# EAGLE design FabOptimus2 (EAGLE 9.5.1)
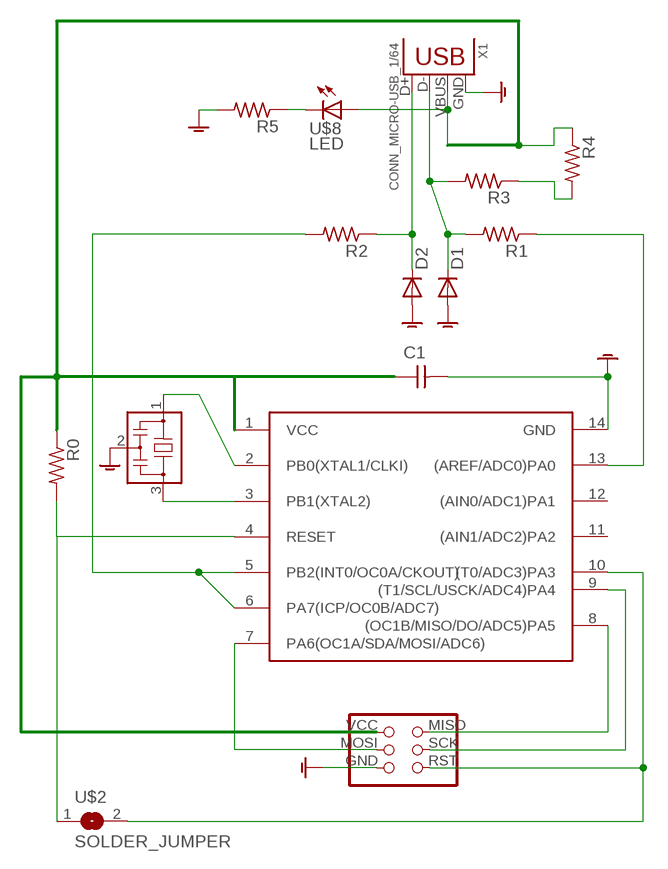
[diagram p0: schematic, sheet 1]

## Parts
C1  CAP-UNPOLARIZEDFAB  [C1206FAB]
D1  DIODESOD123  [SOD123]
D2  DIODESOD123  [SOD123]
IC1  ATTINY44-SSU  [SOIC14_ATTTINY44]
JP1  2X3PINHEADER  [2X3PINHEADER]
R0  RES-US1206FAB  [R1206FAB]
R1  RES-US1206FAB  [R1206FAB]
R2  RES-US1206FAB  [R1206FAB]
R3  RES-US1206FAB  [R1206FAB]
R4  RES-US1206FAB  [R1206FAB]
R5  RES-US1206  [R1206]
U$1  RESONATOR  [EFOBM]
U$2  SOLDER_JUMPER  [SOLDERJUMPER]
U$8  LED  [LED1206]
X1  CONN_MICRO-USB_1/64  [DX4R005HJ5_64]

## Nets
GND: C1.2 D1.ANODE(A) D2.ANODE(A) IC1.14(GND) JP1.GND R5.2 U$1.2 X1.GND
N$1: IC1.2(PB0(XTAL1/CLKI)) U$1.1
N$2: D2.CATHODE(C) R2.1 X1.D+
N$3: IC1.9((T1/SCL/USCK/ADC4)PA4) JP1.SCK
N$4: D1.CATHODE(C) R1.2 R3.2 X1.D-
N$5: IC1.7(PA6(OC1A/SDA/MOSI/ADC6)) JP1.MOSI
N$6: IC1.5(PB2(INT0/OC0A/CKOUT)) IC1.6(PA7(ICP/OC0B/ADC7)) R2.2
N$7: IC1.3(PB1(XTAL2)) U$1.3
N$8: IC1.13((AREF/ADC0)PA0) R1.1
N$9: IC1.8((OC1B/MISO/DO/ADC5)PA5) JP1.MISO
N$10: IC1.10((T0/ADC3)PA3) JP1.RST U$2.2
N$11: IC1.4(RESET) R0.2 U$2.1
N$12: R3.1 R4.2
N$14: R5.1 U$8.2(C)
R4: C1.1 IC1.1(VCC) JP1.VCC R0.1 R4.1 U$8.1(A) X1.VBUS
Unconnected: IC1.11((AIN1/ADC2)PA2) IC1.12((AIN0/ADC1)PA1)

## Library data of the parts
C1 = fab:CAP-UNPOLARIZED
D1 D2 = fab:DIODE: DIODE
IC1 = myFab:ATTINY44
JP1 = myFab:2X3PINHEADER: PIN HEADER
R0 R1-R5 = fab:RES-US: Resistor (US Symbol)
U$1 = fab:RESONATOR
U$2 = myFab:SOLDER_JUMPER
U$8 = fab:LED: LED
X1 = fab:CONN_MICRO-USB: SMD micro USB connector as found in the fablab inventory. Three footprint variants included: original, as described by manufacturer's datasheet for milling with the 1/100" bit for milling with the 1/64" bit Made by Zaerc.

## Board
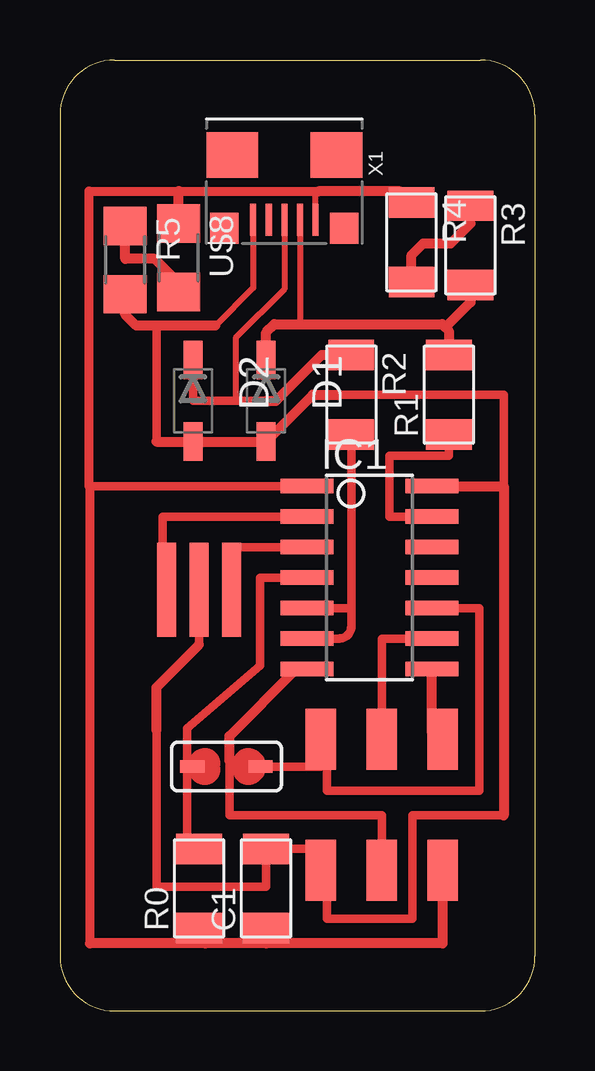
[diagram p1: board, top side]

Size 19.81 x 39.62 mm. Coordinates in mm from the lower left corner, seen from the top.
Outline: 2.29,39.62 17.53,39.62 arc-90 19.81,37.34 19.81,2.29 arc-90 17.53,0 2.29,0 arc-90 0,2.29 0,37.34 arc-90 2.29,39.62
Copper layers (1*16): Top 0.035mm / dielectric 1.5mm / Bottom 0.035mm
Design rules "default *": minimum track width 10mil, minimum drill 24mil, track to track 16mil, track to pad 16mil, pad to pad 16mil, via to via 16mil, smd to smd 16mil, copper to edge 40mil, drill to drill 8mil, minimum pad ring 10mil, minimum via ring 8mil, stop-mask expansion 4mil, vias tented up to drill 0mil, thermal gap 10mil

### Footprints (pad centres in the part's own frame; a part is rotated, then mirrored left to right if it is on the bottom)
C1206FAB = smd 1.27 x 1.905: 1 -1.651,0; 2 1.651,0
SOD123 = smd 1.6 x 0.8: ANODE 1.7,0; CATHODE -1.7,0
SOIC14_ATTTINY44 = smd 2.21 x 0.61: 1 -3.873,3.81; 2 -3.873,2.54; 3 -3.873,1.27; 4 -3.873,0; 5 -3.873,-1.27; 6 -3.873,-2.54; 7 -3.873,-3.81; 8 1.333,-3.81; 9 1.333,-2.54; 10 1.333,-1.27; 11 1.333,0; 12 1.333,1.27; 13 1.333,2.54; 14 1.333,3.81
2X3PINHEADER = smd 2.54 x 1.27: GND -2.54,2.54; MISO 2.92,-2.54; MOSI -2.54,0; RST 2.92,2.54; SCK 2.92,0; VCC -2.54,-2.54
R1206FAB = smd 1.27 x 1.905: 1 -1.651,0; 2 1.651,0
R1206 = smd 1.6 x 1.803: 1 -1.422,0; 2 1.422,0
EFOBM = smd 0.8 x 3.9: 1 -1.35,0; 2 0,0; 3 1.35,0
SOLDERJUMPER = smd 1.016 x 0.508: 1 -2.057,0; 2 0.787,0
LED1206 = smd 1.6 x 1.803: 1 -1.422,0; 2 1.422,0
DX4R005HJ5_64 = smd 0.254 x 1.35: D+ 0,1.6; D- -0.65,1.6; GND 1.3,1.6; ID 0.65,1.6; VBUS -1.3,1.6 | smd 1.2 x 1.3: GND@1 -2.5,1.95; GND@2 2.5,1.95 | smd 2.15 x 1.9: GND@3 -2.175,-1.1; GND@4 2.175,-1.1

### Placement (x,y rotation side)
C1  8.6,5.11 90 top
D1  8.6,25.43 270 top
D2  5.55,25.43 270 top
IC1  14.18,18.06 0 top
JP1  13.42,8.41 90 top
R0  5.8,5.11 90 top
R1  16.22,25.68 90 top
R2  12.15,25.68 270 top
R3  17.12,31.9 270 top
R4  14.66,32.03 270 top
R5  2.72,31.29 270 top
U$1  5.8,17.55 0 top
U$2  7.58,10.19 0 top
U$8  4.95,31.39 270 top
X1  9.36,34.57 180 top

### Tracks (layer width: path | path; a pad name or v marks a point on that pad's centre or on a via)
GND
  Top 0.254: X1.GND 8.06,30.13 6.48,28.56
  Top 0.356: 16.21,21.87 IC1.14 | 18.5,8.15 14.69,8.15 14.69,3.84 11.14,3.84 11.14,4.85 arc90 10.88,5.11 | 4.02,11.71 4.02,5.17 8.6,5.17 C1.2 10.88,6.76 JP1.GND | 18.5,21.87 18.5,25.68 11.64,25.68 | 4.02,23.72 4.02,28.56 | 5.8,15.27 U$1.2
  Top 0.406: 10.88,5.11 JP1.GND | 18.5,8.15 18.5,21.87 16.21,21.87 | 4.02,23.72 D2.ANODE D1.ANODE 10.55,25.68 11.64,25.68 | 4.02,11.71 4.02,13.49 5.8,15.27 | 6.48,28.56 4.02,28.56 3.18,28.56 2.72,29.02 R5.2
N$1
  Top 0.356: IC1.2 4.28,20.6 4.28,17.38 arc-90 U$1.1
N$2
  Top 0.254: X1.D+ 9.36,30.08 7.32,28.04 7.32,25.43
  Top 0.356: D2.CATHODE 5.55,25.43 7.32,25.43 8.6,25.43
  Top 0.406: 8.6,25.43 9.01,25.43 10.91,27.33 R2.1
N$3
  Top 0.356: JP1.SCK 13.42,15.52 IC1.9
N$4
  Top 0.254: D1.CATHODE 8.89,27.12 | X1.D- 10.01,28.64 9.99,28.62
  Top 0.406: D1.CATHODE 8.6,28.27 8.94,28.62 9.99,28.62 15.94,28.62 16.07,28.48 | 16.07,28.48 16.21,28.34 R1.2 | R3.2 17.12,29.53 16.07,28.48
N$5
  Top 0.356: 9.86,14.25 IC1.7 | JP1.MOSI 13.42,8.15 7.07,8.15 7.07,10.44
  Top 0.406: 7.07,10.44 7.07,11.45 9.86,14.25
N$6
  Top 0.356: IC1.5 12.15,16.79 | 12.15,16.79 12.15,16.03 arc-90 11.64,15.52 IC1.6 | R2.2 12.15,16.79
N$7
  Top 0.356: IC1.3 7.07,19.33 7.07,17.63 arc90 U$1.3
N$8
  Top 0.356: IC1.13 13.74,20.6 13.74,23.13 16.21,23.13 R1.1
N$9
  Top 0.406: JP1.MISO 15.52,11.58 IC1.8
N$10
  Top 0.356: IC1.10 17.49,16.79 17.49,9.17 11.14,9.17 11.14,11.07 arc90 JP1.RST 10.88,10.18 U$2.2
N$11
  Top 0.356: IC1.4 8.34,18.06 8.34,14.39 5.29,11.78 5.29,10.41 | 5.29,10.41 5.29,7.26 arc90 R0.2 | 5.29,10.41 arc90 U$2.1
N$12
  Top 0.406: R4.2 14.66,31.49 15.15,31.98 16.3,31.98 17.12,32.8 R3.1
N$14
  Top 0.406: U$8.2 4.95,30.34 3.95,31.34 2.72,31.34 R5.1
R4
  Top 0.254: X1.VBUS 10.66,34.04 10.78,34.15 10.78,34.16
  Top 0.356: R0.1 6.05,2.82 | IC1.1 1.25,21.87 1.21,21.87 | C1.1 8.6,2.82
  Top 0.368: 1.21,21.87 1.21,34.16
  Top 0.381: 1.21,34.16 4.95,34.16 10.78,34.16 | 1.25,2.82 1.25,21.87
  Top 0.406: JP1.VCC 15.96,2.82 8.6,2.82 6.05,2.82 1.25,2.82 | R4.1 14.19,34.15 10.78,34.15 | U$8.1 4.95,34.16

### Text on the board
Labels: USB | R_pullup | C | C | D / 3.3V | D / 3.3V | A | A | 100Ω | 100Ω | 20 / MHz | ATTiny44 | 0Ω | ISP | 10K | 1μF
